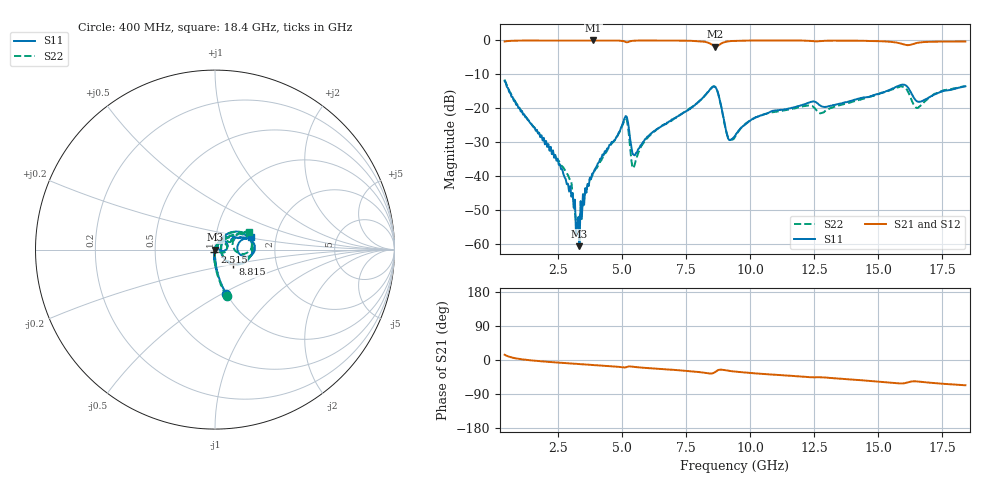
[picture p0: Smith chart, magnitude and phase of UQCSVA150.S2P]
!  Part Number  UQCSVA150  Mounting Orientation: Horizontal
!  Description: Ultra Low ESR Microwave capacitors
!  Application: Coupling, Bypass, Tuning, DC Block
!  Filters, Matching
# GHZ S DB R 50
! Freq  |S11|  S11 Ph  |S21|  S21 Ph  |S12|  S12 Ph  |S22|  S22 Ph
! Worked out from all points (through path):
!   401 points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, 400 MHz to 18.4 GHz, reference 50 ohm
!   highest |S21| = 0.00 dB at 3.865 GHz (marker M1); lowest = -1.8 dB at 8.635 GHz (marker M2)
!   group delay of S21, straight-line fit = 10.7 ps
!   lowest |S11| = -60.7 dB at 3.325 GHz (marker M3), VSWR 1.00, Z = 50.1 + j0.0113 ohm
!   |S11| at or under -10 dB: start of sweep to end of sweep
!   |S22| runs from -54.9 to -11.5 dB; largest |S21 - S12| = 0.026
!   S11 on the Smith chart (normalised r, x): 400 MHz: 0.99, -0.52; 2.515 GHz: 0.99, -0.03; 8.815 GHz: 1.20, -0.20; 18.4 GHz: 1.48, +0.22
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0.4  -11.95 -76.3  -0.29 13.8  -0.08 13.2  -11.52 -75.7
2.515  -36.65 -104.9  -0.01 -7.0  -0.03 -7.7  -35.51 -91.7
2.92  -44.58 -84.5  -0.01 -8.9  -0.04 -9.5  -40.49 -88.8
3.19  -57.13 -25.5  0.00 -10.1  -0.05 -10.6  -53.19 -63.6
3.325  -60.67 7.0  -0.01 -10.7  -0.05 -11.2  -52.01 11.4
3.415  -52.64 24.7  0.00 -11.1  -0.05 -11.5  -49.97 35.8
3.55  -43.53 68.9  -0.01 -11.7  -0.06 -12.1  -44.65 54.7
3.865  -39.11 62.7  0.00 -13.1  -0.05 -13.4  -39.27 63.1
5.08  -23.09 44.2  -0.30 -19.7  -0.33 -19.7  -23.61 31.2
5.44  -33.73 18.9  -0.08 -18.1  -0.10 -18.1  -37.61 25.0
6.43  -25.75 59.0  -0.01 -23.3  -0.01 -23.5  -25.76 59.0
8.635  -13.75 -8.6  -1.79 -31.4  -1.80 -31.2  -13.74 -6.0
8.815  -17.83 -39.1  -1.12 -25.5  -1.15 -25.5  -18.00 -37.1
9.13  -28.88 -20.2  -0.27 -28.1  -0.30 -28.1  -28.51 -15.7
9.4  -28.18 26.8  -0.13 -30.6  -0.14 -30.5  -28.44 29.4
10.345  -22.32 46.8  -0.01 -36.1  0.00 -36.0  -22.30 47.1
12.415  -18.06 34.9  -0.19 -45.6  -0.18 -45.7  -19.32 29.9
12.775  -19.43 26.8  -0.17 -45.6  -0.15 -45.7  -21.40 36.4
15.43  -14.65 20.5  -0.37 -59.5  -0.34 -59.2  -14.78 26.7
16.015  -13.06 0.1  -1.21 -61.3  -1.15 -61.2  -13.81 3.0
16.51  -17.95 -3.6  -0.73 -56.5  -0.66 -56.6  -19.94 12.0
18.4  -13.52 19.6  -0.30 -66.7  -0.27 -66.9  -13.50 28.0
